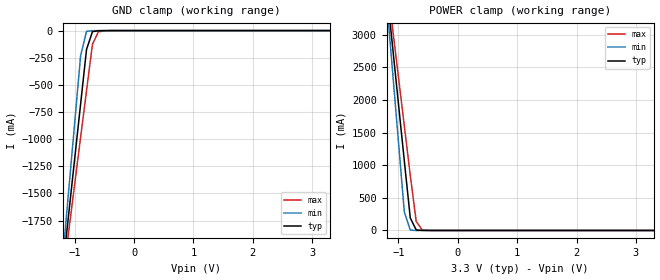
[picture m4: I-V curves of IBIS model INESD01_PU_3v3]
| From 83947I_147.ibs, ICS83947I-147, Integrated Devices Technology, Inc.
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[Model] INESD01_PU_3v3
Model_type   Input
Polarity   Non-Inverting
Vinl = 0.8V
Vinh = 2.0V
|   typ   min   max
C_comp   2pF   1.5pF   2.5pF
|   typ   min   max
[Voltage range]  3.3V   3.15V   3.45V
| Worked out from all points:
|   GND clamp passes 1 mA (typ) near -0.55 V on its own axis
|   POWER clamp passes 1 mA (typ) near -0.61 V on its own axis
[GND_clamp]
|Voltage   I(typ)   I(min)   I(max)
-3.3V     -12.83A    -15.14A    -11.37A
-1.2V     -2.195A    -2.092A    -2.281A
-1.1V     -1.689A    -1.472A    -1.849A
-900mV    -678.5mA   -232.7mA   -984.8mA
-800mV    -174mA     -7.237mA   -553.3mA
-700mV    -9.767mA   -1.114mA   -126.1mA
-600mV    -1.7mA     -240.1uA   -11.15mA
-300mV    -81.66uA   -67.79uA   -163.4uA
3.3V      1.866nA    1.113pA    239.1nA
[POWER_clamp]
|Voltage   I(typ)   I(min)   I(max)
-3.3V     22.38A     26.45A     19.82A
-1.2V     3.723A     3.545A     3.874A
-1.1V     2.836A     2.457A     3.116A
-1V       1.949A     1.369A     2.358A
-900mV    1.063A     281mA      1.601A
-800mV    191.5mA    5.012mA    843.9mA
-700mV    8.032mA    142.2uA    138.3mA
-600mV    607uA      17.63uA    10.62mA
-400mV    16.32uA    7.545uA    335.9uA
3.3V      -71.13uA   -62.11uA   -78.26uA
